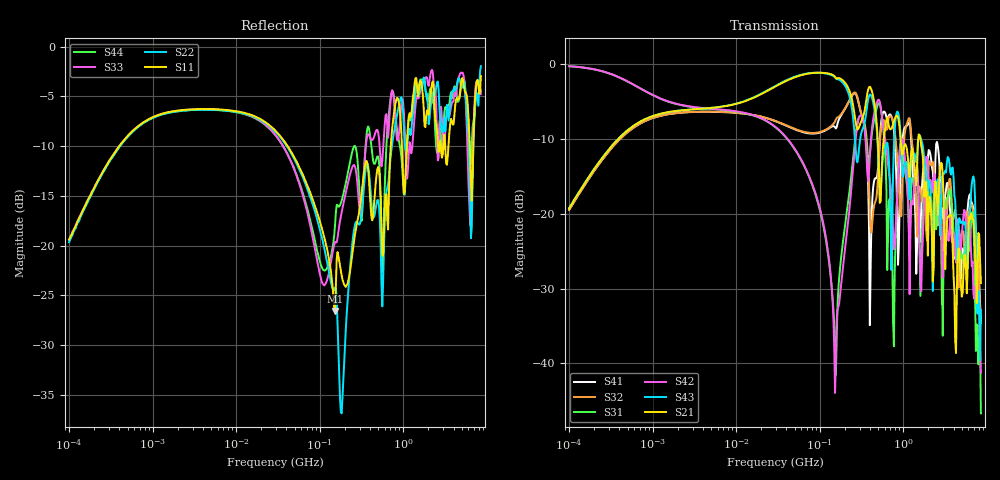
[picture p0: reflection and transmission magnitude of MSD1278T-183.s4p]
# MHz S MA R 50
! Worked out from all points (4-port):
!   498 points, 100 kHz to 8.5 GHz, reference 50 ohm
!   strongest paths, dB at 100 kHz, 1.698 MHz, 29.49 MHz, 500.7 MHz, 8.5 GHz:
!     S21: -19.3, -6.3, -2.9, -11.3, -29.3
!     S43: -19.2, -6.3, -2.9, -12.0, -32.9
!     S42: -0.2, -5.1, -8.3, -4.7, -41.2
!     S31: -0.2, -5.1, -8.4, -5.3, -46.7
!     S32: -19.5, -6.6, -7.6, -14.7, -33.7
!     S41: -19.5, -6.6, -7.6, -13.7, -34.6
!   lowest |S11| = -26.5 dB at 152.7 MHz (marker M1), VSWR 1.10, Z = 53.6 - j3.26 ohm
!   |S11| at or under -10 dB: 41.35 MHz to 708.7 MHz (667.3 MHz wide, 178 % of centre); 3.182 GHz to 3.475 GHz (292.7 MHz wide, 8.79 % of centre); 6.268 GHz to 6.904 GHz (636.7 MHz wide, 9.67 % of centre)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
0.1  0.1076 74.9  0.1084 75.6  0.9731 -6.3  0.1065 -105.0
     0.1084 75.6  0.104 75.5  0.1065 -104.7  0.9742 -6.3
     0.9731 -6.3  0.1065 -104.7  0.1073 75.6  0.1093 75.5
     0.1065 -105.0  0.9742 -6.3  0.1093 75.5  0.1066 76.2
36.21878  0.3419 -46.4  0.7569 7.9  0.3421 -54.5  0.3981 119.1
          0.7569 7.9  0.3379 -49.2  0.3999 116.9  0.3443 -54.0
          0.3421 -54.5  0.3999 116.9  0.3177 -47.9  0.7646 6.5
          0.3981 119.1  0.3443 -54.0  0.7646 6.5  0.3179 -45.4
152.6826  0.04706 -40.2  0.8252 -39.8  0.01226 156.2  0.3798 42.6
          0.8252 -39.8  0.06163 -78.2  0.4162 44.1  0.006329 -128.5
          0.01226 156.2  0.4162 44.1  0.1046 7.9  0.8186 -47.1
          0.3798 42.6  0.006329 -128.5  0.8186 -47.1  0.1274 22.9
500.661  0.2486 -17.1  0.2731 -130.4  0.5453 -66.4  0.2067 -2.6
         0.2731 -130.4  0.1695 -44.4  0.1839 -0.9  0.5804 -52.7
         0.5453 -66.4  0.1839 -0.9  0.3721 -28.7  0.2506 -137.3
         0.2067 -2.6  0.5804 -52.7  0.2506 -137.3  0.2805 -49.4
772.667  0.4603 -39.9  0.4136 -98.9  0.01299 2.7  0.3595 -139.4
         0.4136 -98.9  0.3702 -23.7  0.3918 -124.1  0.05794 -112.7
         0.01299 2.7  0.3918 -124.1  0.5434 -94.7  0.2825 -25.0
         0.3595 -139.4  0.05794 -112.7  0.2825 -25.0  0.5614 -90.0
2159.325  0.61 -165.2  0.1009 92.3  0.1011 127.9  0.2299 130.5
          0.1009 92.3  0.5262 -163.0  0.211 133.6  0.1639 133.4
          0.1011 127.9  0.211 133.6  0.7534 -176.6  0.1175 52.0
          0.2299 130.5  0.1639 133.4  0.1175 52.0  0.6195 173.9
8500  0.712 -36.2  0.03444 -121.1  0.004626 115.8  0.0187 171.9
      0.03444 -121.1  0.7982 -42.4  0.02063 -157.6  0.008677 51.7
      0.004626 115.8  0.02063 -157.6  0.577 -50.9  0.02277 10.8
      0.0187 171.9  0.008677 51.7  0.02277 10.8  0.5986 -50.1
